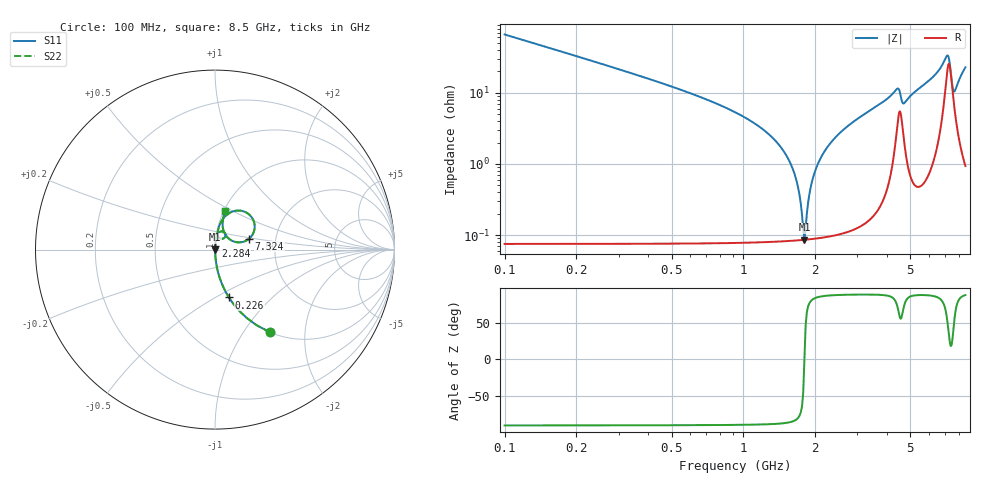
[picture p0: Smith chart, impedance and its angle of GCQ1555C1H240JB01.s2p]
!Murata Part Number: GCQ1555C1H240JB01
!These Parameters are Measured in Series Mode Connection
!Data Generated on Jan 08, 2026
!  o--ll--o
!Port1  Port2
!  o------o
!Operation Temp=25[degC], DC Bias Voltage=0[V]
!Freq. Start=100[MHz] Stop=9[GHz] 401[Steps]
# Hz S RI R 50
!Freq.(Hz) S11(Real) S11(Imag) S21(Real) S21(Imag) S12(Real) S12(Imag) S22(Real) S22(Imag)
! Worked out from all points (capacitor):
!   401 points, 100 MHz to 8.5 GHz, reference 50 ohm
!   read as one part in series: C = 24 pF near 142 MHz
!   lowest |Z| = 85.9 mohm at 1.801 GHz (marker M1)
!   series resonance near 1.8 GHz, so ESL is about 330 pH
!   S11 on the Smith chart (normalised r, x): 100 MHz: 1.00, -1.32; 226 MHz: 1.00, -0.58; 2.284 GHz: 1.00, +0.04; 7.324 GHz: 1.46, +0.19; 8.5 GHz: 1.02, +0.46
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1e8  0.3044 -0.4596  0.6956 0.4596  0.6956 0.4596  0.3044 -0.4596
2.26e8  0.0776 -0.2663  0.9224 0.2663  0.9224 0.2663  0.0776 -0.2663
6.04e8  0.0102 -0.0966  0.9898 0.0966  0.9898 0.0966  0.0102 -0.0966
1.213e9  0.0017 -0.0301  0.9983 0.0301  0.9983 0.0301  0.0017 -0.0301
1.507e9  0.000999 -0.0134  0.999 0.0134  0.999 0.0134  0.000999 -0.0134
1.654e9  0.000878 -0.00638  0.9991 0.00638  0.9991 0.00638  0.000878 -0.00638
1.759e9  0.000854 -0.00175  0.9991 0.00175  0.9991 0.00175  0.000854 -0.00175
1.801e9  0.000857 3.71e-05  0.9991 -3.71e-05  0.9991 -3.71e-05  0.000857 3.71e-05
1.843e9  0.000867 0.00178  0.9991 -0.00178  0.9991 -0.00178  0.000867 0.00178
1.906e9  0.000892 0.00434  0.9991 -0.00434  0.9991 -0.00434  0.000892 0.00434
1.99e9  0.000947 0.00765  0.9991 -0.00765  0.9991 -0.00765  0.000947 0.00765
2.284e9  0.00129 0.0185  0.9987 -0.0185  0.9987 -0.0185  0.00129 0.0185
2.914e9  0.0028 0.0399  0.9972 -0.0399  0.9972 -0.0399  0.0028 0.0399
4.3e9  0.0262 0.0991  0.9738 -0.0991  0.9738 -0.0991  0.0262 0.0991
4.468e9  0.0556 0.0919  0.9444 -0.0919  0.9444 -0.0919  0.0556 0.0919
4.678e9  0.0284 0.0626  0.9716 -0.0626  0.9716 -0.0626  0.0284 0.0626
5.707e9  0.0219 0.1272  0.9781 -0.1272  0.9781 -0.1272  0.0219 0.1272
6.652e9  0.0687 0.1963  0.9313 -0.1963  0.9313 -0.1963  0.0687 0.1963
7.114e9  0.1985 0.1873  0.8015 -0.1873  0.8015 -0.1873  0.1985 0.1873
7.324e9  0.1909 0.0615  0.8091 -0.0615  0.8091 -0.0615  0.1909 0.0615
7.618e9  0.0687 0.069  0.9313 -0.069  0.9313 -0.069  0.0687 0.069
8.5e9  0.0574 0.2131  0.9426 -0.2131  0.9426 -0.2131  0.0574 0.2131
